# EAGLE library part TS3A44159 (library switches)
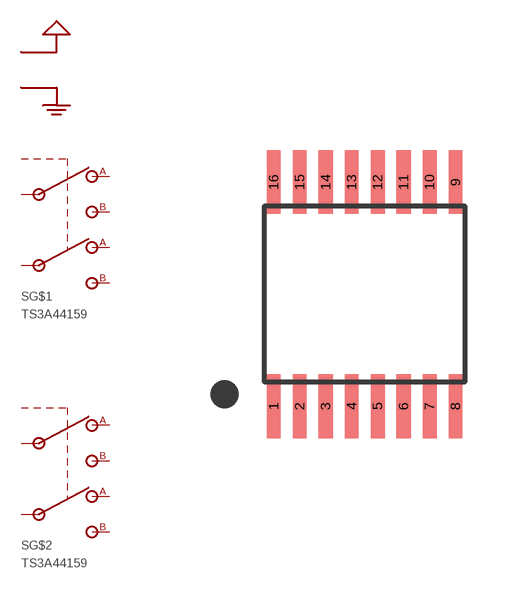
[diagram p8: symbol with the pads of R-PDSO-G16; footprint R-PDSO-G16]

Designator prefix S; gates G$1=DPDT-DIGITAL G$2=DPDT-DIGITAL G$3=PWR

## TS3A44159PWR (DIGIKEY: 296-21915-1-ND)  [R-PDSO-G16]
1  G$1:B0
2  G$1:B
3  G$1:B1
4  G$3:GND
5  G$2:A0
6  G$2:A
7  G$2:A1
8  G$2:CTRL
9  G$2:B0
10  G$2:B
11  G$2:B1
12  G$3:VCC
13  G$1:A0
14  G$1:A
15  G$1:A1
16  G$1:CTRL

## Footprint R-PDSO-G16 (pad centres in mm)
smd 0.35 x 1.6: 1 -2.275,-2.8; 2 -1.625,-2.8; 3 -0.975,-2.8; 4 -0.325,-2.8; 5 0.325,-2.8; 6 0.975,-2.8; 7 1.625,-2.8; 8 2.275,-2.8; 9 2.275,2.8; 10 1.625,2.8; 11 0.975,2.8; 12 0.325,2.8; 13 -0.325,2.8; 14 -0.975,2.8; 15 -1.625,2.8; 16 -2.275,2.8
